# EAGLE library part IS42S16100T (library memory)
512K Words x 16 Bits x 2 Banks (16-MBIT) SYNCHRONOUS DYNAMIC RAM Source: www.issi.com .. IS42S16100.pdf
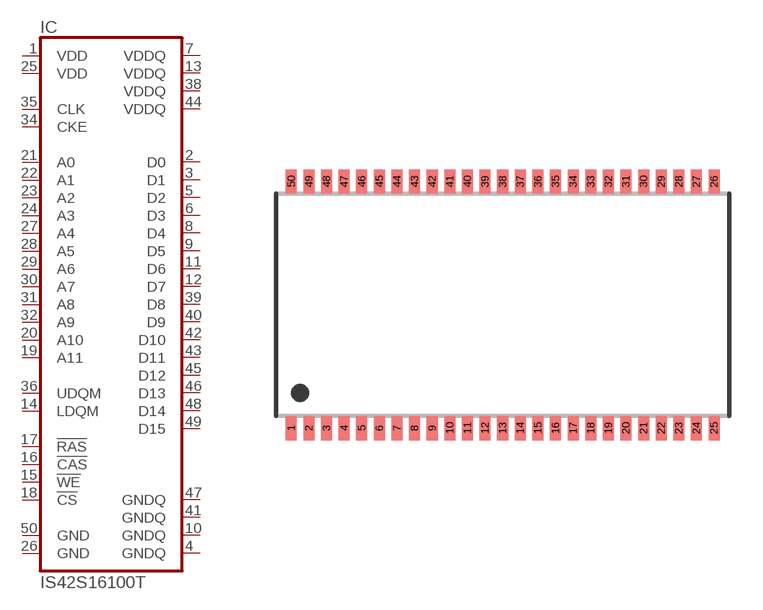
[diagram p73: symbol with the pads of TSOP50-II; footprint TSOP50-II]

Designator prefix IC

## IS42S16100T  [TSOP50-II]
1  VDD  pwr
2  D0
3  D1
4  GNDQ  pwr
5  D2
6  D3
7  VDDQ  pwr
8  D4
9  D5
10  GNDQ  pwr
11  D6
12  D7
13  VDDQ  pwr
14  LDQM  in
15  !WE  in
16  !CAS  in
17  !RAS  in
18  !CS  in
19  A11  in
20  A10  in
21  A0  in
22  A1  in
23  A2  in
24  A3  in
25  VDD  pwr
26  GND  pwr
27  A4  in
28  A5  in
29  A6  in
30  A7  in
31  A8  in
32  A9  in
34  CKE  in
35  CLK  in
36  UDQM  in
38  VDDQ  pwr
39  D8
40  D9
41  GNDQ  pwr
42  D10
43  D11
44  VDDQ  pwr
45  D12
46  D13
47  GNDQ  pwr
48  D14
49  D15
50  GND  pwr

## Footprint TSOP50-II (pad centres in mm)
TSOP 50 Type II Source: www.issi.com .. IS42S16100.pdf
smd 0.5 x 1.1: 1 -9.6,-5.6; 2 -8.8,-5.6; 3 -8,-5.6; 4 -7.2,-5.6; 5 -6.4,-5.6; 6 -5.6,-5.6; 7 -4.8,-5.6; 8 -4,-5.6; 9 -3.2,-5.6; 10 -2.4,-5.6; 11 -1.6,-5.6; 12 -0.8,-5.6; 13 0,-5.6; 14 0.8,-5.6; 15 1.6,-5.6; 16 2.4,-5.6; 17 3.2,-5.6; 18 4,-5.6; 19 4.8,-5.6; 20 5.6,-5.6; 21 6.4,-5.6; 22 7.2,-5.6; 23 8,-5.6; 24 8.8,-5.6; 25 9.6,-5.6; 26 9.6,5.6; 27 8.8,5.6; 28 8,5.6; 29 7.2,5.6; 30 6.4,5.6; 31 5.6,5.6; 32 4.8,5.6; 33 4,5.6; 34 3.2,5.6; 35 2.4,5.6; 36 1.6,5.6; 37 0.8,5.6; 38 0,5.6; 39 -0.8,5.6; 40 -1.6,5.6; 41 -2.4,5.6; 42 -3.2,5.6; 43 -4,5.6; 44 -4.8,5.6; 45 -5.6,5.6; 46 -6.4,5.6; 47 -7.2,5.6; 48 -8,5.6; 49 -8.8,5.6; 50 -9.6,5.6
